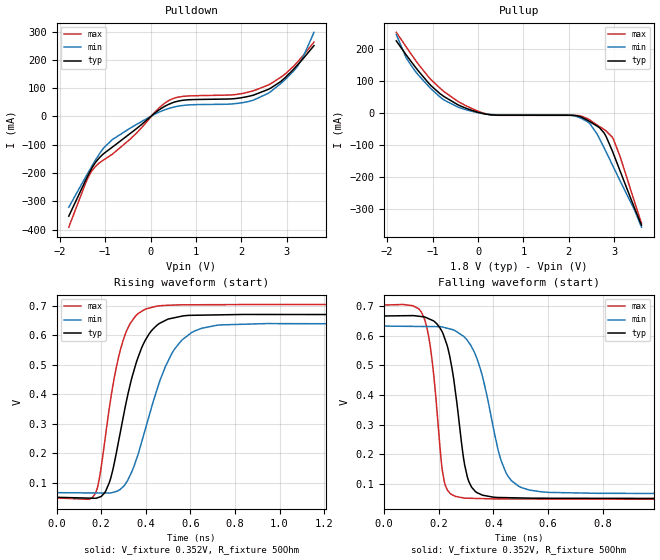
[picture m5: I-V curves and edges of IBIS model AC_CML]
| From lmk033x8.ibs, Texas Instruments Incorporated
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[Model]   AC_CML
Model_type   Output
Polarity   Non-Inverting
Vmeas = 0.9
Vref = 1.8
Cref = 15pF
Rref = 50
|   typ   min   max
|   (nom PVT)   (fast PVT)   (slow PVT)
C_comp   0.989p   0.973p   0.998p
|C_comp (ON state)   0.989p   0.973p   0.998p
|C_comp (OFF state)   0.989p   0.973p   0.998p
| Where   nom PVT is  Nominal Process, 1.8V, 27C
|   Fast PVT is Strong Process, 1.9V, -40C
|   Slow PVT is Weak Process, 1.7V, 125C
[Voltage Range]   1.8   1.7   1.9
[Temperature Range]   27   125   -40
[Pullup Reference]   1.8   1.7   1.9
[Pulldown Reference]   0   0   -0
[Power Clamp Reference]   1.8   1.7   1.9
[GND Clamp Reference]   0   0   0
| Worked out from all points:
|   slope of the pulldown table from 0 to 0.27 V, typ, clamps not added: 8.31 ohm
|   slope of the pullup table from 0 to 0.27 V, typ, clamps not added: 35.3 ohm
|   falling waveform, V_fixture 0.352V, R_fixture 50Ohm: 20-80 % time 56ps typ, 86.7ps min, 41.3ps max; typ from 0.667 V to 0.051 V
|   rising waveform, V_fixture 0.352V, R_fixture 50Ohm: 20-80 % time 114ps typ, 147ps min, 89.7ps max; typ from 0.051 V to 0.667 V
[Pulldown]
|   Voltage   I(typ)   I(min)   I(max)
-1.8V     -352.6mA   -321.1mA   -391.4mA
-1.438V   -228.9mA   -216.7mA   -239.5mA
-1.282V   -179.8mA   -173.2mA   -190.1mA
-1.044V   -133.3mA   -113.9mA   -155mA
-838.8mV  -108.4mA   -81.82mA   -133.4mA
311.4mV   35.4mA     23.15mA    46.42mA
705.6mV   56.82mA    38.54mA    70.52mA
2.034V    66.91mA    48.83mA    81.36mA
2.59V     95.3mA     81.38mA    110.6mA
2.871V    123.7mA    116.5mA    138.6mA
3.244V    182.8mA    178.8mA    193.2mA
3.6V      250.1mA    297.2mA    262.8mA
[Pullup]
|   Voltage   I(typ)   I(min)   I(max)
-1.8V     227mA      247mA      253.8mA
-1.579V   182mA      172.6mA    207.2mA
-1.082V   93.41mA    83.36mA    112.4mA
-747mV    51.98mA    41.31mA    67.47mA
-142.2mV  9.261mA    6.229mA    15.09mA
316.8mV   -5.425mA   -4.344mA   -5.74mA
2.104V    -6.755mA   -8.155mA   -6.832mA
2.461V    -26.35mA   -32.26mA   -21.35mA
2.677V    -45.75mA   -80.1mA    -42.15mA
2.817V    -72.09mA   -120.3mA   -55.3mA
2.979V    -126mA     -168.2mA   -80.78mA
3.6V      -351.3mA   -357.5mA   -345.9mA
[Ramp]
R_load = 50
|   typ   min   max
dV/dt_r   0.369883/1.13329e-10   0.339961/1.45548e-10   0.393339/8.93715e-11
dV/dt_f   0.369883/5.58136e-11   0.339961/8.66612e-11   0.393339/4.13014e-11
[Falling Waveform]
V_fixture = 0.352V
V_fixture_min = 0.346V
V_fixture_max = 0.365V
R_fixture = 50Ohm
C_fixture = 0F
|   Time   V(typ)   V(min)   V(max)
0s        667.1mV    632.9mV    704mV
146.4ps   664.1mV    631.6mV    660.3mV
175.9ps   652.7mV    631.3mV    516.3mV
211ps     616.4mV    630.3mV    162.2mV
249.2ps   486.5mV    621.4mV    63.62mV
291.5ps   182.6mV    598.1mV    52.78mV
333.8ps   74.91mV    537.2mV    51.45mV
444.8ps   54.1mV     140.2mV    49.55mV
574.3ps   52.13mV    73.81mV    49.4mV
6.7ns     50.61mV    66.34mV    48.48mV
[Rising Waveform]
V_fixture = 0.352V
V_fixture_min = 0.346V
V_fixture_max = 0.365V
R_fixture = 50Ohm
C_fixture = 0F
|   Time   V(typ)   V(min)   V(max)
0s        50.61mV    66.34mV    48.48mV
159.3ps   47.56mV    65.46mV    48.48mV
186ps     49.53mV    65.31mV    91.42mV
218.1ps   68.58mV    65.13mV    250.7mV
306ps     349.3mV    92.6mV     598.9mV
380.9ps   555.9mV    235.7mV    680.4mV
445.3ps   630.1mV    403mV      698mV
561.3ps   664.5mV    583.1mV    703.1mV
735.4ps   669.1mV    635mV      703.6mV
6.7ns     667.1mV    632.9mV    704mV
